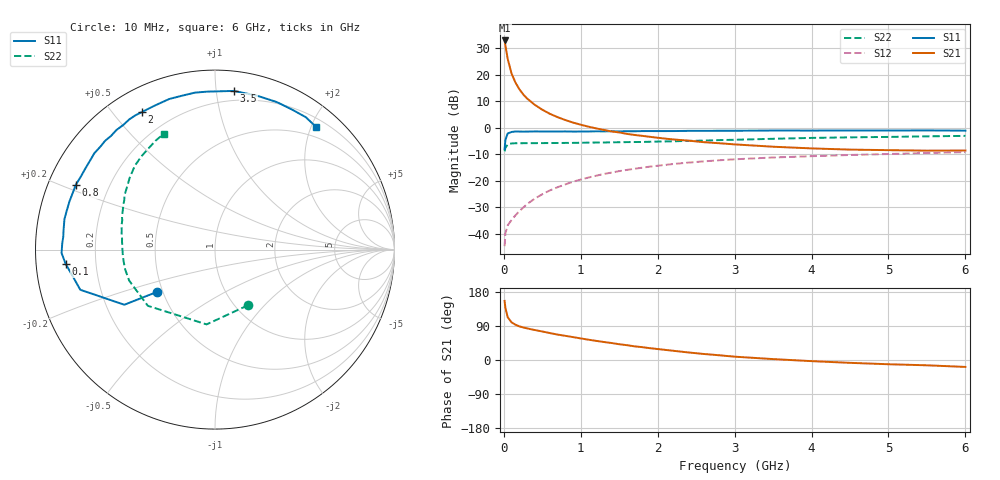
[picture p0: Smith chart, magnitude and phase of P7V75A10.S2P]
! SIEMENS Small Signal Semiconductors
! BFP196
! Si NPN RF Bipolar Junction Transistor in SOT143
! VCE = 0.75 V  IC = 100 mA
! Common Emitter S-Parameters:  May  1996
# GHz  S  MA  R  50
!  f  S11  S21  S12  S22
! GHz  MAG  ANG  MAG  ANG  MAG  ANG  MAG  ANG
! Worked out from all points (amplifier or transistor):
!   36 points, 10 MHz to 6 GHz, reference 50 ohm
!   highest |S21| = 32.9 dB at 10 MHz (marker M1)
!   |S21| within 3 dB of that: start of sweep to 26.88 MHz
!   unconditionally stable (mu >= 1): start of sweep to 16.92 MHz; 155.8 MHz to end of sweep
!   at 250 MHz: K = 1.19, MAG = 18.8 dB, |S12| = -30.1 dB
!   at 1.4 GHz: K = 1.24, MAG = 4.8 dB, |S12| = -16.9 dB
!   at 6 GHz: K = 1.09, MAG = -1.6 dB, |S12| = -9.2 dB
!   S11 on the Smith chart (normalised r, x): 10 MHz: 0.46, -0.26; 100 MHz: 0.09, -0.05; 800 MHz: 0.08, +0.22; 2 GHz: 0.10, +0.60; 3.5 GHz: 0.13, +1.12; 6 GHz: 0.33, +2.08
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0.01  0.4004 -143.9  44.29 155.9  0.0059 58.6  0.3605 -59.5
0.02  0.5915 -148.7  35.88 137.9  0.0103 51.1  0.4194 -96.4
0.05  0.7831 -163.4  19.92 113.0  0.0146 41.2  0.4881 -140.1
0.1  0.8361 -174.6  10.59 99.3  0.0183 46.4  0.5085 -160.2
0.15  0.8551 -178.7  7.172 93.2  0.0224 51.7  0.5125 -167.5
0.2  0.8518 177.7  5.399 88.9  0.0267 56.9  0.5126 -171.4
0.25  0.8485 175.1  4.296 86.0  0.0313 59.2  0.5138 -174.1
0.3  0.8503 173.1  3.596 83.5  0.0364 61.6  0.5143 -175.9
0.4  0.8558 168.6  2.728 79.2  0.0462 64.3  0.5149 -178.6
0.5  0.8541 165.5  2.196 75.3  0.0561 65.4  0.5162 179.4
0.6  0.8542 161.7  1.834 71.0  0.0664 65.3  0.5169 177.8
0.7  0.8532 157.9  1.587 67.0  0.0763 64.9  0.5183 176.3
0.8  0.8554 155.1  1.401 63.8  0.0861 63.7  0.5201 175.0
1.1  0.8542 145.0  1.053 53.6  0.1158 59.9  0.5265 171.1
1.5  0.8584 132.4  0.819 41.6  0.1531 53.4  0.5356 166.2
2  0.868 118.0  0.65 28.9  0.1934 44.5  0.5514 159.7
2.2  0.8698 112.6  0.605 24.4  0.2082 41.1  0.5578 157.1
2.8  0.8817 97.3  0.513 12.5  0.245 31.2  0.588 149.0
3.5  0.8903 83.2  0.441 2.4  0.2764 20.3  0.6218 139.8
4.5  0.8912 67.3  0.389 -7.5  0.3082 7.7  0.6621 128.2
5.5  0.8945 55.6  0.372 -14.0  0.3359 -3.1  0.6915 118.5
6  0.8857 50.4  0.374 -18.3  0.3483 -8.9  0.7059 113.7
